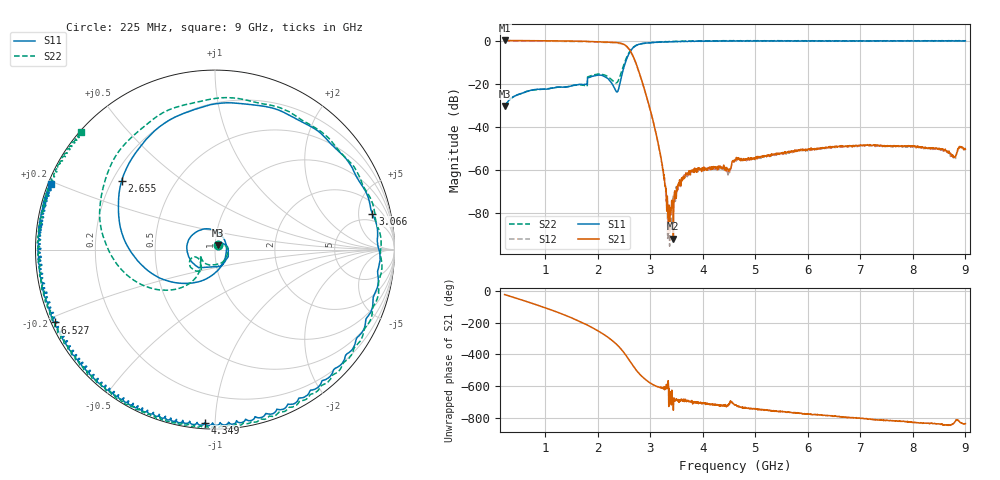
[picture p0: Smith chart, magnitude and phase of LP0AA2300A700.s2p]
!Agilent Technologies,E8358A,US41080443,A.07.50.56
!Agilent E8358A: A.07.50.56
!Date: Wednesday, August 31, 2016 08:46:45
!Correction: S11(Full 2 Port(1,2))
!S21(Full 2 Port(1,2))
!S12(Full 2 Port(1,2))
!S22(Full 2 Port(1,2))
!S2P File: Measurements: S11, S21, S12, S22:
# Hz S  dB  R 50
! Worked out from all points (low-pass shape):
!   1601 points, 225 MHz to 9 GHz, reference 50 ohm
!   highest |S21| = 0.04 dB at 225 MHz (marker M1); lowest = -92.0 dB at 3.439 GHz (marker M2)
!   |S21| within 3 dB of the highest: start of sweep to 2.562 GHz
!   lowest |S11| = -30.4 dB at 225 MHz (marker M3), VSWR 1.06, Z = 51.4 + j2.71 ohm
!   |S11| at or under -10 dB: start of sweep to 2.528 GHz
!   |S22| runs from -30.5 to 0.0 dB; largest |S21 - S12| = 0.023
!   S11 on the Smith chart (normalised r, x): 225 MHz: 1.03, +0.05; 2.655 GHz: 0.24, +0.31; 3.066 GHz: 3.45, +7.24; 4.349 GHz: 0.03, -0.94; 6.527 GHz: 0.01, -0.22; 9 GHz: 0.01, +0.19
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2.25e8  -30.40 60.7  0.04 -23.6  -0.14 -23.3  -30.49 61.0
6.363281e8  -23.64 23.5  -0.05 -66.8  -0.24 -66.6  -23.74 16.0
9.70875e8  -22.56 -4.9  -0.12 -104.0  -0.30 -103.7  -22.56 -26.6
1.382203e9  -21.68 -42.0  -0.21 -154.5  -0.40 -154.2  -21.52 -86.4
1.689328e9  -20.35 -76.4  -0.33 161.8  -0.50 162.1  -20.59 -135.1
2.095172e9  -16.32 151.1  -0.65 88.9  -0.83 89.1  -15.77 -150.4
2.24325e9  -19.06 96.5  -0.76 54.6  -0.95 54.9  -17.74 -161.1
2.385844e9  -23.19 -30.1  -1.02 13.0  -1.21 13.3  -18.73 -134.2
2.544891e9  -8.80 -156.5  -2.57 -51.0  -2.74 -50.8  -8.06 -145.8
2.654578e9  -3.78 143.5  -6.36 -104.7  -6.53 -104.5  -3.56 165.3
2.830078e9  -1.47 70.7  -17.94 -176.5  -18.12 -176.2  -1.49 89.7
3.065906e9  -0.92 12.9  -38.62 125.3  -38.85 126.4  -0.91 22.1
3.153656e9  -0.72 -2.5  -48.25 113.8  -48.35 113.6  -0.67 4.7
3.340125e9  -0.55 -27.4  -82.61 153.5  -87.10 103.4  -0.46 -22.9
3.438844e9  -0.57 -38.5  -92.00 -32.6  -79.57 22.7  -0.45 -34.6
3.680156e9  -0.36 -59.3  -61.40 28.0  -61.59 28.3  -0.24 -55.3
4.34925e9  -0.30 -93.4  -58.70 -4.6  -58.93 -1.1  -0.17 -88.1
4.6125e9  -0.26 -102.8  -55.23 1.4  -55.82 1.1  -0.13 -96.7
6.076828e9  -0.12 -143.5  -50.16 -61.2  -50.36 -59.4  -0.08 -139.4
6.526547e9  -0.16 -155.6  -49.17 -70.7  -49.69 -71.7  -0.09 -153.9
7.541156e9  -0.25 179.6  -49.03 -98.2  -49.11 -98.6  -0.18 173.0
9e9  -0.14 158.0  -50.47 -117.0  -50.70 -116.3  -0.07 138.9
